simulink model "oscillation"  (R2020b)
settings: Solver=FixedStepAuto  StartTime=0.0  StopTime=20  FixedStep=0.02  RelTol=1e-3
libraries: sldrtlib x1

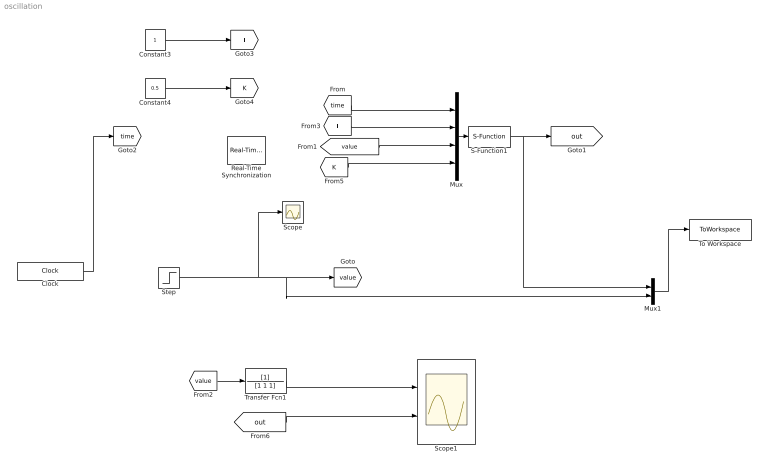
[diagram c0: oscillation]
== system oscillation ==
  Clock : Clock
  Constant3 : Constant
  Constant4 : Constant  Value=0.5
  Mux : Mux
  Mux1 : Mux  Inputs=2
  Real-Time Synchronization : sldrtlib/Real-Time Synchronization  SampleTime=0.02  MaxMissedTicks=inf  ShowMissedTicks=off  YieldWhenWaiting=off
  S-Function1 : S-Function  FunctionName=modbusComoscillation  SFunctionDeploymentMode=off  EnableBusSupport=off
  Scope : Scope
  Scope1 : Scope  NumInputPorts=2
  Step : Step  SampleTime=0
  To Workspace : ToWorkspace  VariableName=simout  SampleTime=-1
  Transfer Fcn1 : TransferFcn  Denominator=[1 1 1]
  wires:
  S-Function1/1 -> Mux1/1, [out]
  Clock/1 -> [time]
  [out] -> Scope1/2
  [value] -> Mux/3
  Mux/1 -> S-Function1/1
  [time] -> Mux/1
  [T] -> Mux/2
  Constant3/1 -> [T]
  Constant4/1 -> [K]
  [K] -> Mux/4
  Step/1 -> Scope/1, Mux1/2, [value]
  [value] -> Transfer Fcn1/1
  Transfer Fcn1/1 -> Scope1/1
  Mux1/1 -> To Workspace/1
